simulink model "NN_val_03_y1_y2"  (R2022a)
settings: Solver=VariableStepAuto  StartTime=0.0  StopTime=300  RelTol=1e-3
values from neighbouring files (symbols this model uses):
  C = 6.3000e-04    (= 0.00063)    [maglev_init.m]
  g = 9.80    (= 9.8)    [maglev_init.m]
  K = 1.0e+03 * [-2.4567   -0.1235    0.0237]    [maglev_init.m]
  L1 = 0.6000    (= 0.6)    [maglev_init.m]
  m = 0.0300    (= 0.03)    [maglev_init.m]
  mpert = 0    [maglev_init.m]
  R = 45    [maglev_init.m]
  Ts = 0.005    [maglev_init.m]    (also in train_net.m)
  x1_0 = 0.1    [maglev_init.m]
  x1_d = 0.05    [maglev_init.m]
  x2_0 = 0    [maglev_init.m]
  x2_d = 0    [maglev_init.m]
  x3_0 = 0.2    [maglev_init.m]
undefined symbols (not defined in the file or in its folder): magnitude
libraries: neural x32

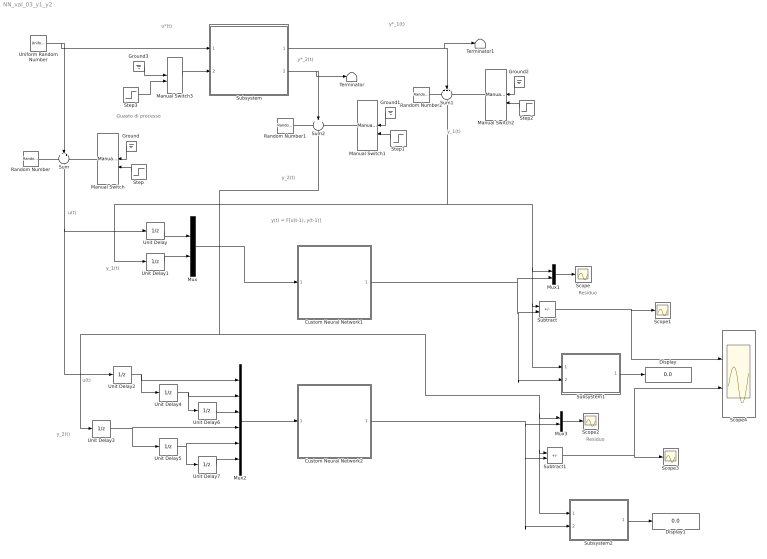
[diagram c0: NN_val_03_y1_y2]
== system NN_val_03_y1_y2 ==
  note: Residuo
  note: y(t) = F[u(t-1), y(t-1)]
  note: y_2(t)
  note: y*_1(t)
  note: u(t)
  note: y*_2(t)
  note: y_1(t)
  note: u*(t)
  note: Guasto di processo
  note: Residuo
  note: y_1(t)
  note: u(t)
  note: y_2(t)
  Custom Neural Network1 : Subsystem
      mask help: Custom Neural Network
  Custom Neural Network2 : Subsystem
      mask help: Custom Neural Network
  Display : Display
  Display1 : Display
  Ground{,1..3} (4 alike) : Ground
  Manual Switch : ManualSwitch  CurrentSetting=0
  Manual Switch1 : ManualSwitch
  Manual Switch2 : ManualSwitch
  Manual Switch3 : ManualSwitch
  Mux : Mux  Inputs=2
  Mux1 : Mux  Inputs=2
  Mux2 : Mux  Inputs=6
  Mux3 : Mux  Inputs=2
  Random Number : RandomNumber  Variance=1e-9  Seed=1  SampleTime=Ts
  Random Number1 : RandomNumber  Variance=1e-6  Seed=3  SampleTime=Ts
  Random Number2 : RandomNumber  Variance=1e-9  Seed=2  SampleTime=Ts
  Scope{,1..3} (4 alike) : Scope
  Scope4 : Scope  NumInputPorts=2
  Step : Step  Time=150  SampleTime=0
  Step1 : Step  Time=150  SampleTime=0
  Step2 : Step  Time=150  SampleTime=0
  Step3 : Step  Time=15  After=2*R  SampleTime=0
  Subsystem : Subsystem
  Subsystem1 : Subsystem
  Subsystem2 : Subsystem
  Subtract : Sum  Inputs=+-
  Subtract1 : Sum  Inputs=+-
  Sum : Sum  Inputs=+++
  Sum1 : Sum  Inputs=+++
  Sum2 : Sum  Inputs=+++
  Terminator : Terminator
  Terminator1 : Terminator
  Uniform Random Number : UniformRandomNumber  Minimum=x1_d*0.9  Maximum=x1_d*1.1  Seed=1  SampleTime=0.5
  Unit Delay{,1..7} (8 alike) : UnitDelay  SampleTime=Ts  HasFrameUpgradeWarning=on
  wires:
  Subsystem/1(Out1) -> Terminator1/1, Sum1/2
  Subsystem/2(Out2) -> Terminator/1, Sum2/2
  Random Number/1 -> Sum/1
  Manual Switch/1 -> Sum/3
  Manual Switch2/1 -> Sum1/3
  Manual Switch1/1 -> Sum2/3
  Random Number1/1 -> Sum2/1
  Ground/1 -> Manual Switch/1
  Step/1 -> Manual Switch/2
  Ground1/1 -> Manual Switch1/1
  Step1/1 -> Manual Switch1/2
  Random Number2/1 -> Sum1/1
  Ground2/1 -> Manual Switch2/1
  Step2/1 -> Manual Switch2/2
  Manual Switch3/1 -> Subsystem/2(fs)
  Ground3/1 -> Manual Switch3/1
  Uniform Random Number/1 -> Subsystem/1(u), Sum/2
  Step3/1 -> Manual Switch3/2
  Sum/1 -> Unit Delay2/1, Unit Delay/1
  Unit Delay/1 -> Mux/1
  Unit Delay1/1 -> Mux/2
  Mux/1 -> Custom Neural Network1/1(Input)
  Custom Neural Network1/1(Output) -> Mux1/2, Subsystem1/2(y_prev), Subtract/2
  Subtract/1 -> Scope4/1, Scope1/1
  Mux1/1 -> Scope/1
  Sum1/1 -> Subsystem1/1(y_mis), Subtract/1, Mux1/1, Unit Delay1/1
  Subsystem1/1(VAF%) -> Display/1
  Mux2/1 -> Custom Neural Network2/1(Input)
  Subtract1/1 -> Scope4/2, Scope3/1
  Custom Neural Network2/1(Output) -> Subsystem2/2(y_prev), Subtract1/2, Mux3/2
  Mux3/1 -> Scope2/1
  Subsystem2/1(VAF%) -> Display1/1
  Sum2/1 -> Subsystem2/1(y_mis), Subtract1/1, Mux3/1, Unit Delay3/1
  Unit Delay2/1 -> Unit Delay4/1, Mux2/1
  Unit Delay4/1 -> Unit Delay6/1, Mux2/2
  Unit Delay3/1 -> Unit Delay5/1, Mux2/4
  Unit Delay5/1 -> Unit Delay7/1, Mux2/5
  Unit Delay6/1 -> Mux2/3
  Unit Delay7/1 -> Mux2/6

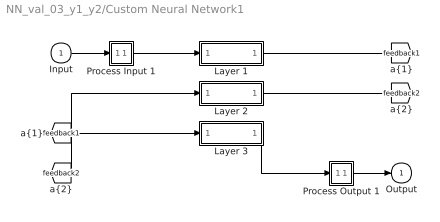
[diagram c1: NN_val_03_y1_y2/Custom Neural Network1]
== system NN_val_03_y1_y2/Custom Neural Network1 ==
  Input : Inport  PortDimensions=2  SampleTime=0.005
  Layer 1 : Subsystem
  Layer 2 : Subsystem
  Layer 3 : Subsystem
  Process Input 1 : Subsystem
  Process Output 1 : Subsystem
  Output : Outport  InitialOutput=0
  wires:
  Layer 3/1("a{3}") -> Process Output 1/1(a)
  [feedback2] -> Layer 3/1("a{2} ")
  Layer 2/1("a{2}") -> [feedback2]
  [feedback1] -> Layer 2/1("a{1} ")
  Layer 1/1("a{1}") -> [feedback1]
  Process Input 1/1(p) -> Layer 1/1("p{1}")
  Process Output 1/1(y) -> Output/1
  Input/1 -> Process Input 1/1(x)

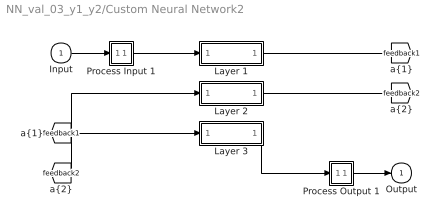
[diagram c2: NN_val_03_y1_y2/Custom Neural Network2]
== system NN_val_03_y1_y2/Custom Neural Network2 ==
  Input : Inport  PortDimensions=6  SampleTime=0.005
  Layer 1 : Subsystem
  Layer 2 : Subsystem
  Layer 3 : Subsystem
  Process Input 1 : Subsystem
  Process Output 1 : Subsystem
  Output : Outport  InitialOutput=0
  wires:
  Input/1 -> Process Input 1/1(x)
  Process Output 1/1(y) -> Output/1
  Process Input 1/1(p) -> Layer 1/1("p{1}")
  Layer 1/1("a{1}") -> [feedback1]
  [feedback1] -> Layer 2/1("a{1} ")
  Layer 2/1("a{2}") -> [feedback2]
  [feedback2] -> Layer 3/1("a{2} ")
  Layer 3/1("a{3}") -> Process Output 1/1(a)

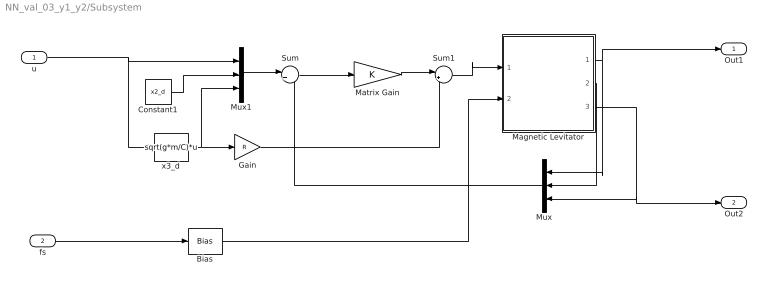
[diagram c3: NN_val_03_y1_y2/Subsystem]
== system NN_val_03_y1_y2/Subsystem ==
  u : Inport
  fs : Inport  Port=2
  Bias : Bias  Bias=R
  Constant1 : Constant  Value=x2_d
  Gain : Gain  Gain=R
  Magnetic Levitator : Subsystem  mask{m=m+mpert, R=R, L1=L1, C=C, g=g}
      mask prompts: m "ball's mass (m)"; R "Electromagnet's resistance (R)"; L1 "Electromagnet's inductance (L1)"; C "Magnetic force constant (C)"; g "Gravitational acceleration (g)"
  Matrix Gain : Gain  Gain=K  Multiplication=Matrix(K*u)  SaturateOnIntegerOverflow=on
  Mux : Mux  Inputs=3
  Mux1 : Mux  Inputs=3
  Sum : Sum  Inputs=|+-  InputSameDT=on  SaturateOnIntegerOverflow=on
  Sum1 : Sum  Inputs=|++  InputSameDT=on  SaturateOnIntegerOverflow=on
  x3_d : Fcn  Expr=sqrt(g*m/C)*u
  Out1 : Outport
  Out2 : Outport  Port=2
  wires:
  u/1 -> x3_d/1, Mux1/1
  Magnetic Levitator/2(x2) -> Mux/2
  x3_d/1 -> Mux1/3, Gain/1
  Mux1/1 -> Sum/1
  Gain/1 -> Sum1/2
  Mux/1 -> Sum/2
  Constant1/1 -> Mux1/2
  Sum/1 -> Matrix Gain/1
  Sum1/1 -> Magnetic Levitator/1(u)
  Magnetic Levitator/1(x1) -> Out1/1, Mux/1
  Magnetic Levitator/3(x3) -> Out2/1, Mux/3
  Matrix Gain/1 -> Sum1/1
  Bias/1 -> Magnetic Levitator/2(fs)
  fs/1 -> Bias/1

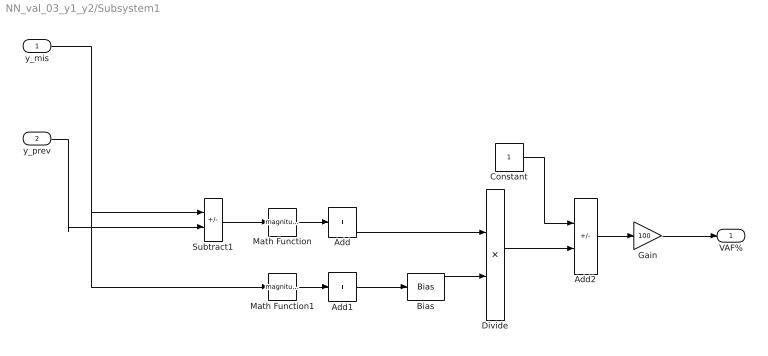
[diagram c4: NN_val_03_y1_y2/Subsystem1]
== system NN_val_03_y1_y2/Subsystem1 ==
  y_mis : Inport
  y_prev : Inport  Port=2
  Add : Sum  Inputs=+
  Add1 : Sum  Inputs=+
  Add2 : Sum  Inputs=+-
  Bias : Bias  Bias=1e-7
  Constant : Constant
  Divide : Product  Inputs=*/
  Gain : Gain  Gain=100
  Math Function : Math  Operator=magnitude^2
  Math Function1 : Math  Operator=magnitude^2
  Subtract1 : Sum  Inputs=+-
  VAF% : Outport
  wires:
  Add2/1 -> Gain/1
  Math Function/1 -> Add/1
  Bias/1 -> Divide/2
  y_mis/1 -> Math Function1/1, Subtract1/1
  Add1/1 -> Bias/1
  Math Function1/1 -> Add1/1
  Subtract1/1 -> Math Function/1
  Constant/1 -> Add2/1
  Divide/1 -> Add2/2
  Add/1 -> Divide/1
  y_prev/1 -> Subtract1/2
  Gain/1 -> VAF%/1

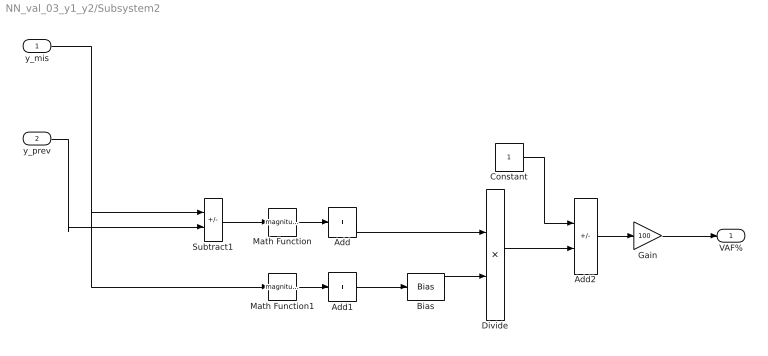
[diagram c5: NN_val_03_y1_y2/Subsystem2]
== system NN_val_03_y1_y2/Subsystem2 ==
  y_mis : Inport
  y_prev : Inport  Port=2
  Add : Sum  Inputs=+
  Add1 : Sum  Inputs=+
  Add2 : Sum  Inputs=+-
  Bias : Bias  Bias=1e-7
  Constant : Constant
  Divide : Product  Inputs=*/
  Gain : Gain  Gain=100
  Math Function : Math  Operator=magnitude^2
  Math Function1 : Math  Operator=magnitude^2
  Subtract1 : Sum  Inputs=+-
  VAF% : Outport
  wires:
  Add2/1 -> Gain/1
  Math Function/1 -> Add/1
  Bias/1 -> Divide/2
  y_mis/1 -> Math Function1/1, Subtract1/1
  Add1/1 -> Bias/1
  Math Function1/1 -> Add1/1
  Subtract1/1 -> Math Function/1
  Constant/1 -> Add2/1
  Divide/1 -> Add2/2
  Add/1 -> Divide/1
  y_prev/1 -> Subtract1/2
  Gain/1 -> VAF%/1

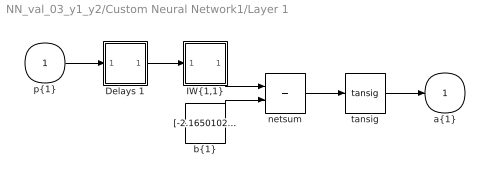
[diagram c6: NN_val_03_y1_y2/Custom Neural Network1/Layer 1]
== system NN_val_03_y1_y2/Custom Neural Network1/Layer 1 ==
  "p{1}" : Inport  PortDimensions=2  SampleTime=0.005
  Delays 1 : Subsystem
  "IW{1,1}" : Subsystem
  "b{1}" : Constant  Value=[-2.165010232984565075042837634100578725337982177734375;-0.99018084463472033629471980020753107964992523193359375]
  netsum : Sum  Inputs=2  InputSameDT=on  SaturateOnIntegerOverflow=on
  tansig : neural/Transfer Functions/tansig
  "a{1}" : Outport  InitialOutput=[0;0]
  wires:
  tansig/1 -> "a{1}"/1
  netsum/1 -> tansig/1
  "b{1}"/1 -> netsum/2
  "IW{1,1}"/1("iz{1,1}") -> netsum/1
  Delays 1/1("pd{1,1}") -> "IW{1,1}"/1("pd{1,1}")
  "p{1}"/1 -> Delays 1/1("p{1}")

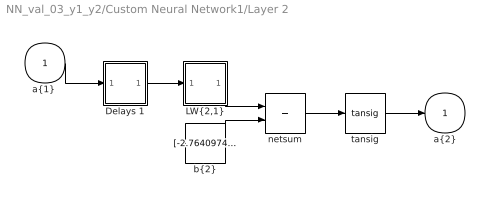
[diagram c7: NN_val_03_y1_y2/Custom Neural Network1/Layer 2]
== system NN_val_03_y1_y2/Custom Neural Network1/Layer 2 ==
  "a{1} " : Inport  PortDimensions=2  SampleTime=0.005
  Delays 1 : Subsystem
  "LW{2,1}" : Subsystem
  "b{2}" : Constant  Value=[-2.76409742947160541604034733609296381473541259765625;0.91391405324340713178798978333361446857452392578125;-0.79693396570784413857069239384145475924015045166015625;2.83340357653886432132139816530980169773101806640625]
  netsum : Sum  Inputs=2  InputSameDT=on  SaturateOnIntegerOverflow=on
  tansig : neural/Transfer Functions/tansig
  "a{2}" : Outport  InitialOutput=[0;0;0;0]
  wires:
  tansig/1 -> "a{2}"/1
  netsum/1 -> tansig/1
  "b{2}"/1 -> netsum/2
  "LW{2,1}"/1("lz{2,1}") -> netsum/1
  Delays 1/1("pd{2,1}") -> "LW{2,1}"/1("ad{2,1}")
  "a{1} "/1 -> Delays 1/1("p{2}")

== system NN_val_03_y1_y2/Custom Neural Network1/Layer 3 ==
  "a{2} " : Inport  PortDimensions=4  SampleTime=0.005
  Delays 1 : Subsystem
  "LW{3,2}" : Subsystem
  "b{3}" : Constant  Value=0.2010605623167778244209102922468446195125579833984375
  netsum : Sum  Inputs=2  InputSameDT=on  SaturateOnIntegerOverflow=on
  purelin : neural/Transfer Functions/purelin
  "a{3}" : Outport  InitialOutput=0
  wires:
  purelin/1 -> "a{3}"/1
  netsum/1 -> purelin/1
  "b{3}"/1 -> netsum/2
  "LW{3,2}"/1("lz{3,2}") -> netsum/1
  Delays 1/1("pd{3,2}") -> "LW{3,2}"/1("ad{3,2}")
  "a{2} "/1 -> Delays 1/1("p{3}")

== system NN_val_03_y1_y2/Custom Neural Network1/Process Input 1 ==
  x : Inport  PortDimensions=2  SampleTime=0.005
  p : Outport  PortDimensions=2  SampleTime=0.005
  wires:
  x/1 -> p/1

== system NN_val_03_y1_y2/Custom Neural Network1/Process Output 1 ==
  a : Inport  PortDimensions=1  SampleTime=0.005
  y : Outport  PortDimensions=1  SampleTime=0.005
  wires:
  a/1 -> y/1

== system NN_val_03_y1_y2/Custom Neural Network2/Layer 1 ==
  "p{1}" : Inport  PortDimensions=6  SampleTime=0.005
  Delays 1 : Subsystem
  "IW{1,1}" : Subsystem
  "b{1}" : Constant  Value=[2.149296792410499090664188770460896193981170654296875;-1.26887349894557832641339700785465538501739501953125;3.373069580518730514739900172571651637554168701171875;-1.7998848449207380806313949506147764623165130615234375;1.2392816118853933193832972392556257545948028564453125;0.81691378138732062552662682719528675079345703125]
  netsum : Sum  Inputs=2  InputSameDT=on  SaturateOnIntegerOverflow=on
  tansig : neural/Transfer Functions/tansig
  "a{1}" : Outport  InitialOutput=[0;0;0;0;0;0]
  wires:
  "p{1}"/1 -> Delays 1/1("p{1}")
  Delays 1/1("pd{1,1}") -> "IW{1,1}"/1("pd{1,1}")
  "IW{1,1}"/1("iz{1,1}") -> netsum/1
  "b{1}"/1 -> netsum/2
  netsum/1 -> tansig/1
  tansig/1 -> "a{1}"/1

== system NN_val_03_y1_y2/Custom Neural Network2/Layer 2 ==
  "a{1} " : Inport  PortDimensions=6  SampleTime=0.005
  Delays 1 : Subsystem
  "LW{2,1}" : Subsystem
  "b{2}" : Constant  Value=[-2.370217449210205273857354768551886081695556640625;-1.29906795532936403247958878637291491031646728515625;1.1720512795939292960412103639100678265094757080078125;1.08189049869129316761018344550393521785736083984375;-0.81222582000211962505176188642508350312709808349609375;0.26111327945252360560601800898439250886440277099609375;-0.2195796660176075054682343079548445530235767364501953125;-0.2526395828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
  netsum : Sum  Inputs=2  InputSameDT=on  SaturateOnIntegerOverflow=on
  tansig : neural/Transfer Functions/tansig
  "a{2}" : Outport  InitialOutput=[0;0;0;0;0;0;0;0;0;0;0;0]
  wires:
  "a{1} "/1 -> Delays 1/1("p{2}")
  Delays 1/1("pd{2,1}") -> "LW{2,1}"/1("ad{2,1}")
  "LW{2,1}"/1("lz{2,1}") -> netsum/1
  "b{2}"/1 -> netsum/2
  netsum/1 -> tansig/1
  tansig/1 -> "a{2}"/1

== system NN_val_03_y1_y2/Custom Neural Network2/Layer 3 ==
  "a{2} " : Inport  PortDimensions=12  SampleTime=0.005
  Delays 1 : Subsystem
  "LW{3,2}" : Subsystem
  "b{3}" : Constant  Value=0.152701582306567329450075476415804587304592132568359375
  netsum : Sum  Inputs=2  InputSameDT=on  SaturateOnIntegerOverflow=on
  purelin : neural/Transfer Functions/purelin
  "a{3}" : Outport  InitialOutput=0
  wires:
  "a{2} "/1 -> Delays 1/1("p{3}")
  Delays 1/1("pd{3,2}") -> "LW{3,2}"/1("ad{3,2}")
  "LW{3,2}"/1("lz{3,2}") -> netsum/1
  "b{3}"/1 -> netsum/2
  netsum/1 -> purelin/1
  purelin/1 -> "a{3}"/1

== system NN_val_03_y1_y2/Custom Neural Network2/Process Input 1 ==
  x : Inport  PortDimensions=6  SampleTime=0.005
  p : Outport  PortDimensions=6  SampleTime=0.005
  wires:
  x/1 -> p/1

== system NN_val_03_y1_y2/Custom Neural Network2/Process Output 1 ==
  a : Inport  PortDimensions=1  SampleTime=0.005
  y : Outport  PortDimensions=1  SampleTime=0.005
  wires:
  a/1 -> y/1

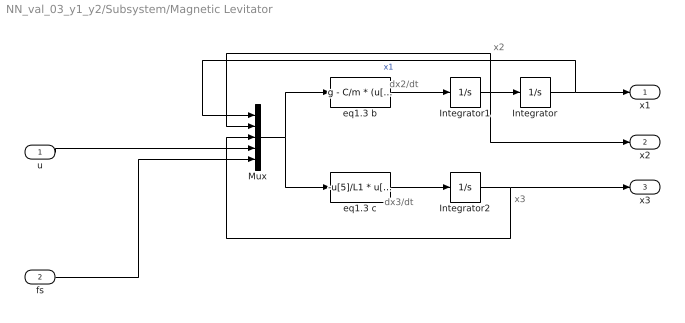
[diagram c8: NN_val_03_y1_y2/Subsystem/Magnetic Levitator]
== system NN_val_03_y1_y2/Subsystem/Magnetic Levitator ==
  note: x2
  note: x3
  note: dx2/dt
  note: dx3/dt
  u : Inport
  fs : Inport  Port=2
  Integrator : Integrator  InitialCondition=x1_0
  Integrator1 : Integrator  InitialCondition=x2_0
  Integrator2 : Integrator  InitialCondition=x3_0
  Mux : Mux  Inputs=5
  eq1.3 b : Fcn  Expr=g - C/m * (u[3] / u[1])^2
  eq1.3 c : Fcn  Expr=-u[5]/L1 * u[3] + (2*C)/L1 * ( u[2] * u[3] / u[1]^2 ) + 1/L1 * u[4]
  x1 : Outport
  x2 : Outport  Port=2
  x3 : Outport  Port=3
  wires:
  eq1.3 b/1 -> Integrator1/1
  Integrator1/1 -> Integrator/1, Mux/2, x2/1
  eq1.3 c/1 -> Integrator2/1
  Mux/1 -> eq1.3 b/1, eq1.3 c/1
  Integrator/1 -> Mux/1, x1/1  "x1"
  Integrator2/1 -> Mux/3, x3/1
  u/1 -> Mux/4
  fs/1 -> Mux/5

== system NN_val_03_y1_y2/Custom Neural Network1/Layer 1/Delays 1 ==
  "p{1}" : Inport  PortDimensions=2  SampleTime=0.005
  mux : Mux  Inputs=1
  "pd{1,1}" : Outport
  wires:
  mux/1 -> "pd{1,1}"/1
  "p{1}"/1 -> mux/1

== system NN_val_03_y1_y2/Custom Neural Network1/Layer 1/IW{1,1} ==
  "pd{1,1}" : Inport  PortDimensions=2  SampleTime=0.005
  "IW{1,1}(1,:)'" : Constant  Value=[46.38752532641807846403025905601680278778076171875;-30.02020716206245509738437249325215816497802734375]
  "IW{1,1}(2,:)'" : Constant  Value=[50.408506029134514392353594303131103515625;28.00458439829532153453328646719455718994140625]
  Mux : Mux  Inputs=2
  dotprod1 : neural/Weight Functions/dotprod
  dotprod2 : neural/Weight Functions/dotprod
  "iz{1,1}" : Outport
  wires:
  Mux/1 -> "iz{1,1}"/1
  dotprod2/1 -> Mux/2
  "IW{1,1}(2,:)'"/1 -> dotprod2/1
  dotprod1/1 -> Mux/1
  "pd{1,1}"/1 -> dotprod2/2, dotprod1/2
  "IW{1,1}(1,:)'"/1 -> dotprod1/1

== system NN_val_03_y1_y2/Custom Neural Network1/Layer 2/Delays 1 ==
  "p{2}" : Inport  PortDimensions=2  SampleTime=0.005
  mux : Mux  Inputs=1
  "pd{2,1}" : Outport
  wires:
  mux/1 -> "pd{2,1}"/1
  "p{2}"/1 -> mux/1

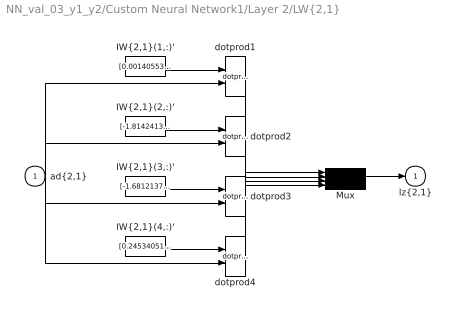
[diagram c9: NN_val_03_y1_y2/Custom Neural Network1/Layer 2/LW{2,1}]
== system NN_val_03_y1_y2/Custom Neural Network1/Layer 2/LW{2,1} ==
  "ad{2,1}" : Inport  PortDimensions=2  SampleTime=0.005
  "IW{2,1}(1,:)'" : Constant  Value=[0.001405533007920074795027431946436990983784198760986328125;2.76441434699151766807290186989121139049530029296875]
  "IW{2,1}(2,:)'" : Constant  Value=[-1.8142413042354241792253333187545649707317352294921875;2.12830136073460085555097975884564220905303955078125]
  "IW{2,1}(3,:)'" : Constant  Value=[-1.6812137832937150694334604850155301392078399658203125;-2.2096304124726291462366134510375559329986572265625]
  "IW{2,1}(4,:)'" : Constant  Value=[0.245340519136751533668672209387295879423618316650390625;2.76382363851122736519982936442829668521881103515625]
  Mux : Mux
  dotprod{1..4} (4 alike) : neural/Weight Functions/dotprod
  "lz{2,1}" : Outport
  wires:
  Mux/1 -> "lz{2,1}"/1
  dotprod4/1 -> Mux/4
  "IW{2,1}(4,:)'"/1 -> dotprod4/1
  dotprod3/1 -> Mux/3
  "IW{2,1}(3,:)'"/1 -> dotprod3/1
  dotprod2/1 -> Mux/2
  "IW{2,1}(2,:)'"/1 -> dotprod2/1
  dotprod1/1 -> Mux/1
  "ad{2,1}"/1 -> dotprod4/2, dotprod3/2, dotprod2/2, dotprod1/2
  "IW{2,1}(1,:)'"/1 -> dotprod1/1

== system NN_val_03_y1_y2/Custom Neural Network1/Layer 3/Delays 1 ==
  "p{3}" : Inport  PortDimensions=4  SampleTime=0.005
  mux : Mux  Inputs=1
  "pd{3,2}" : Outport
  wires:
  mux/1 -> "pd{3,2}"/1
  "p{3}"/1 -> mux/1

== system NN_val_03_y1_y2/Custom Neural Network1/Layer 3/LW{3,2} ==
  "ad{3,2}" : Inport  PortDimensions=4  SampleTime=0.005
  "IW{3,2}(1,:)'" : Constant  Value=[0.483295609205659226770279701668187044560909271240234375;0.356104986175123150449195463806972838938236236572265625;0.2319393811096205626487432027715840376913547515869140625;-0.2873034152097859728058892869739793241024017333984375]
  Mux : Mux  Inputs=1
  dotprod1 : neural/Weight Functions/dotprod
  "lz{3,2}" : Outport
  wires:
  Mux/1 -> "lz{3,2}"/1
  dotprod1/1 -> Mux/1
  "ad{3,2}"/1 -> dotprod1/2
  "IW{3,2}(1,:)'"/1 -> dotprod1/1

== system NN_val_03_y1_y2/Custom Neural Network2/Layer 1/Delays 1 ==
  "p{1}" : Inport  PortDimensions=6  SampleTime=0.005
  mux : Mux  Inputs=1
  "pd{1,1}" : Outport
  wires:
  "p{1}"/1 -> mux/1
  mux/1 -> "pd{1,1}"/1

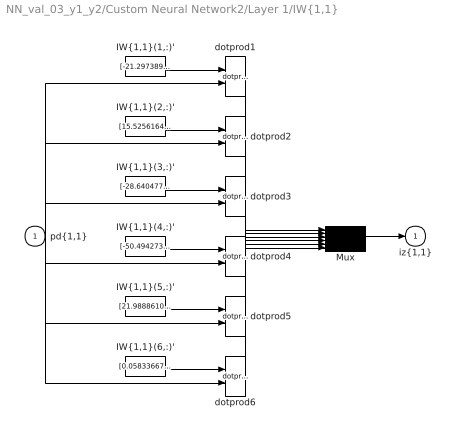
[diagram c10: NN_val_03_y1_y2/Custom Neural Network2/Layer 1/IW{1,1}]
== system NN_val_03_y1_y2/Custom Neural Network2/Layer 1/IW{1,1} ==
  "pd{1,1}" : Inport  PortDimensions=6  SampleTime=0.005
  "IW{1,1}(1,:)'" : Constant  Value=[-21.297389866221227094911228050477802753448486328125;-2.3197865287881231921573998988606035709381103515625;10.463116681280354214322869665920734405517578125;-1.407953418367536624344893425586633384227752685546875;-0.0273185259189663888490517962281955988146364688873291015625;0.67540635506435020563031912388396449387073516845703125]
  "IW{1,1}(2,:)'" : Constant  Value=[15.525616434729609949272344238124787807464599609375;31.36198248157794665758046903647482395172119140625;-24.1252158957646543058217503130435943603515625;0.42313518615797607314021888669230975210666656494140625;-1.0089243874362854302972891673562116920948028564453125;0.10282448271384451998766706992682884447276592254638671875]
  "IW{1,1}(3,:)'" : Constant  Value=[-28.6404775999519216611588490195572376251220703125;10.4745812406206173506006962270475924015045166015625;-24.618714143935829241627288865856826305389404296875;-0.2694353902983610549171089587616734206676483154296875;-1.3866256520797402007616483388119377195835113525390625;-0.941566025450506050020749171380884945392608642578125]
  "IW{1,1}(4,:)'" : Constant  Value=[-50.4942736078991600834342534653842449188232421875;12.468918615817475625817678519524633884429931640625;41.21628720942863566278901998884975910186767578125;0.69524481179556507637329332283115945756435394287109375;0.462307720479153305692676667604246176779270172119140625;0.20544418889201587763437828471069224178791046142578125]
  "IW{1,1}(5,:)'" : Constant  Value=[21.988861062388249223431557766161859035491943359375;32.448750549283204236417077481746673583984375;-42.7550546486075973007245920598506927490234375;0.2975376630584574133564501607907004654407501220703125;-0.71466427493176076790604156485642306506633758544921875;-0.1046345373215911978004299953681766055524349212646484375]
  "IW{1,1}(6,:)'" : Constant  Value=[0.05833667244539410268178158958107815124094486236572265625;26.786850030293596347519269329495728015899658203125;-0.88655409354315273251501139384345151484012603759765625;-0.372604184685911776764299929709522984921932220458984375;0.570511991997245448970943471067585051059722900390625;0.78888488637986797780143888303427956998348236083984375]
  Mux : Mux  Inputs=6
  dotprod{1..6} (6 alike) : neural/Weight Functions/dotprod
  "iz{1,1}" : Outport
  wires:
  "IW{1,1}(1,:)'"/1 -> dotprod1/1
  "pd{1,1}"/1 -> dotprod1/2, dotprod2/2, dotprod3/2, dotprod4/2, dotprod5/2, dotprod6/2
  dotprod1/1 -> Mux/1
  "IW{1,1}(2,:)'"/1 -> dotprod2/1
  dotprod2/1 -> Mux/2
  "IW{1,1}(3,:)'"/1 -> dotprod3/1
  dotprod3/1 -> Mux/3
  "IW{1,1}(4,:)'"/1 -> dotprod4/1
  dotprod4/1 -> Mux/4
  "IW{1,1}(5,:)'"/1 -> dotprod5/1
  dotprod5/1 -> Mux/5
  "IW{1,1}(6,:)'"/1 -> dotprod6/1
  dotprod6/1 -> Mux/6
  Mux/1 -> "iz{1,1}"/1

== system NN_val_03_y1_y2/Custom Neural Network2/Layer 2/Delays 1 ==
  "p{2}" : Inport  PortDimensions=6  SampleTime=0.005
  mux : Mux  Inputs=1
  "pd{2,1}" : Outport
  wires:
  "p{2}"/1 -> mux/1
  mux/1 -> "pd{2,1}"/1

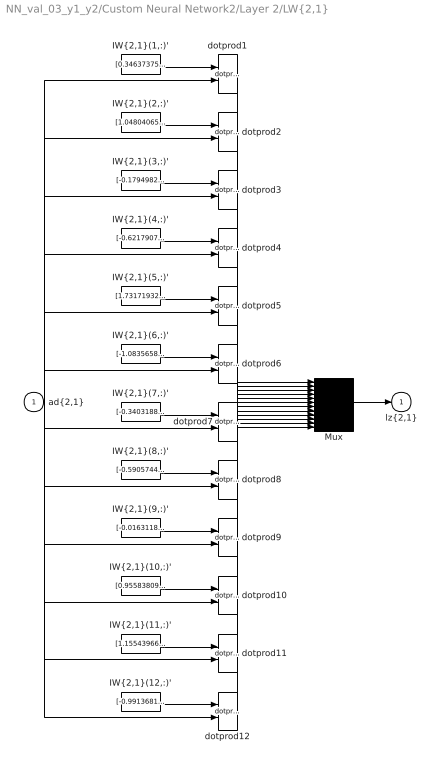
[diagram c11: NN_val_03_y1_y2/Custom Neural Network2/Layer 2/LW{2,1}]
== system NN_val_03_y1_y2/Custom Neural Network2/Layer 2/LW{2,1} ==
  "ad{2,1}" : Inport  PortDimensions=6  SampleTime=0.005
  "IW{2,1}(1,:)'" : Constant  Value=[0.346373757912341873055339647180517204105854034423828125;-0.2914178947601067104500316418125294148921966552734375;-0.90597743139947073398587917836266569793224334716796875;1.50312136755843450686143114580772817134857177734375;-0.150271271091694413879480407558730803430080413818359375;-0.504186126836226211622715709381736814975738525390625]
  "IW{2,1}(10,:)'" : Constant  Value=[0.95583809296900812402242308962740935385227203369140625;-0.97321641546175075010438604294904507696628570556640625;0.2105687367377131469226014814921654760837554931640625;1.416797014452133129935873512295074760913848876953125;0.50214744109140763139720320396008901298046112060546875;0.391547240235185445289545214109239168465137481689453125]
  "IW{2,1}(11,:)'" : Constant  Value=[1.1554396640415613983776665918412618339061737060546875;-1.1758748846940585419673652722849510610103607177734375;0.906524966028687817498621370759792625904083251953125;-0.86328074737005666694500405355938710272312164306640625;-0.07053561671683002132215989377073128707706928253173828125;-0.385546370984425956773833377155824564397335052490234375]
  "IW{2,1}(12,:)'" : Constant  Value=[-0.9913681158276010929597532594925723969936370849609375;-0.370197958430602824808630657571484334766864776611328125;-0.380379946040483307712065652594901621341705322265625;-1.2661701305059349653703293370199389755725860595703125;-0.85067615036158372721075693334569223225116729736328125;0.86380227357225025652809335952042602002620697021484375]
  "IW{2,1}(2,:)'" : Constant  Value=[1.0480406569195819255213564247242175042629241943359375;-0.032225615330172242833928208938232273794710636138916015625;0.033349743287474163666583848453228711150586605072021484375;-0.9382948494795251281885839489405043423175811767578125;1.918293996919582244942148463451303541660308837890625;0.263617470931204189721341890617622993886470794677734375]
  "IW{2,1}(3,:)'" : Constant  Value=[-0.1794982211917084402585942370933480560779571533203125;-0.226467397813474413670320473102037794888019561767578125;-0.626958449505879311658418373554013669490814208984375;0.90557642200395249698630095736007206141948699951171875;0.61460017346421469408568327708053402602672576904296875;-1.7313981117898009642885881476104259490966796875]
  "IW{2,1}(4,:)'" : Constant  Value=[-0.62179073115412120120737426987034268677234649658203125;0.638437883435837516543642777833156287670135498046875;1.6341099504011775689349406093242578208446502685546875;0.4651689742987976661225957286660559475421905517578125;-1.06525896844737832935834376257844269275665283203125;0.290107319833826038379953615731210447847843170166015625]
  "IW{2,1}(5,:)'" : Constant  Value=[1.731719323641687680037648533470928668975830078125;0.05072293275272664325736826640422805212438106536865234375;1.10031886997622674329022629535757005214691162109375;0.63340761893549935024338992661796510219573974609375;-0.73238221309725382024424789051408879458904266357421875;-0.7920435521580955207099350445787422358989715576171875]
  "IW{2,1}(6,:)'" : Constant  Value=[-1.08356589642600820155848850845359265804290771484375;-0.83242781762173689852346569750807248055934906005859375;-1.174895059756197124301024814485572278499603271484375;0.381005898791108077450218161175143904983997344970703125;-0.0243528332688808558936788273285856121219694614410400390625;-0.32987572701089462601231616645236499607563018798828125]
  "IW{2,1}(7,:)'" : Constant  Value=[-0.34031881448398360046070365569903515279293060302734375;-0.443082234154181520136006611210177652537822723388671875;0.63988055034879354199262024849303998053073883056640625;0.96398613286192647020556023562676273286342620849609375;1.5420040770015486231159229646436870098114013671875;0.17806016914458722144587454749853350222110748291015625]
  "IW{2,1}(8,:)'" : Constant  Value=[-0.59057448285311486824156190778012387454509735107421875;-1.5077531755249824474418574027367867529392242431640625;-0.42815527408358267091870175136136822402477264404296875;-1.0564391425448020900290657664299942553043365478515625;-0.52947707639394858691872514100396074354648590087890625;-0.5083005429354836568478503977530635893344879150390625]
  "IW{2,1}(9,:)'" : Constant  Value=[-0.016311887838726717159243406740642967633903026580810546875;1.4301833842254791928638724129996262490749359130859375;-0.3066682999396288522575559909455478191375732421875;-0.93466816782568129529096268015564419329166412353515625;1.1503857867310822715722906650626100599765777587890625;-0.489533727957992770285500228055752813816070556640625]
  Mux : Mux  Inputs=12
  dotprod{1..12} (12 alike) : neural/Weight Functions/dotprod
  "lz{2,1}" : Outport
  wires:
  "IW{2,1}(1,:)'"/1 -> dotprod1/1
  "ad{2,1}"/1 -> dotprod1/2, dotprod2/2, dotprod3/2, dotprod4/2, dotprod5/2, dotprod6/2, dotprod7/2, dotprod8/2, dotprod9/2, dotprod10/2, dotprod11/2, dotprod12/2
  dotprod1/1 -> Mux/1
  "IW{2,1}(2,:)'"/1 -> dotprod2/1
  dotprod2/1 -> Mux/2
  "IW{2,1}(3,:)'"/1 -> dotprod3/1
  dotprod3/1 -> Mux/3
  "IW{2,1}(4,:)'"/1 -> dotprod4/1
  dotprod4/1 -> Mux/4
  "IW{2,1}(5,:)'"/1 -> dotprod5/1
  dotprod5/1 -> Mux/5
  "IW{2,1}(6,:)'"/1 -> dotprod6/1
  dotprod6/1 -> Mux/6
  "IW{2,1}(7,:)'"/1 -> dotprod7/1
  dotprod7/1 -> Mux/7
  "IW{2,1}(8,:)'"/1 -> dotprod8/1
  dotprod8/1 -> Mux/8
  "IW{2,1}(9,:)'"/1 -> dotprod9/1
  dotprod9/1 -> Mux/9
  "IW{2,1}(10,:)'"/1 -> dotprod10/1
  dotprod10/1 -> Mux/10
  "IW{2,1}(11,:)'"/1 -> dotprod11/1
  dotprod11/1 -> Mux/11
  "IW{2,1}(12,:)'"/1 -> dotprod12/1
  dotprod12/1 -> Mux/12
  Mux/1 -> "lz{2,1}"/1

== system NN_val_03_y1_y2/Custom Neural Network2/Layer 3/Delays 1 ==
  "p{3}" : Inport  PortDimensions=12  SampleTime=0.005
  mux : Mux  Inputs=1
  "pd{3,2}" : Outport
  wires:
  "p{3}"/1 -> mux/1
  mux/1 -> "pd{3,2}"/1

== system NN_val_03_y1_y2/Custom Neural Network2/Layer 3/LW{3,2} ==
  "ad{3,2}" : Inport  PortDimensions=12  SampleTime=0.005
  "IW{3,2}(1,:)'" : Constant  Value=[0.55661098872920800051389278451097197830677032470703125;-0.0229932797396699729886027085967725724913179874420166015625;0.337956691755495308715495639262371696531772613525390625;0.72271245642480563819987082752049900591373443603515625;-1.4583592858545564308059283575857989490032196044921875;0.11717415122095097002041796940829954110085964202880859375;1.115390990750681821097600732173305004835128784179687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
  Mux : Mux  Inputs=1
  dotprod1 : neural/Weight Functions/dotprod
  "lz{3,2}" : Outport
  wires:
  "IW{3,2}(1,:)'"/1 -> dotprod1/1
  "ad{3,2}"/1 -> dotprod1/2
  dotprod1/1 -> Mux/1
  Mux/1 -> "lz{3,2}"/1
